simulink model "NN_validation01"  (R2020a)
settings: Solver=ode45  StartTime=0.0  StopTime=2000  RelTol=1e-3  EnableMultiTasking=on
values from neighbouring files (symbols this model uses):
  Ts = 0.2    [init_model.m]
libraries: neural x26

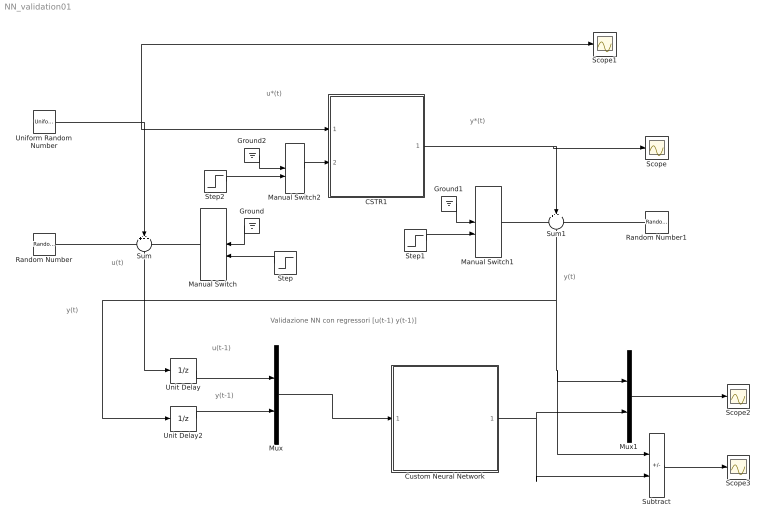
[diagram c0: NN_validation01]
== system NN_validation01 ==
  note: u(t)
  note: u*(t)
  note: y(t)
  note: y*(t)
  note: Validazione NN con regressori [u(t-1) y(t-1)]
  note: u(t-1)
  note: y(t)
  note: y(t-1)
  CSTR1 : Subsystem
  Custom Neural Network : Subsystem
      mask help: Custom Neural Network
  Ground : Ground
  Ground1 : Ground
  Ground2 : Ground
  Manual Switch : ManualSwitch
  Manual Switch1 : ManualSwitch
  Manual Switch2 : ManualSwitch
  Mux : Mux  Inputs=2
  Mux1 : Mux  Inputs=2
  Random Number : RandomNumber  Variance=0.0001  Seed=1  SampleTime=Ts
  Random Number1 : RandomNumber  Variance=0.0005  Seed=2  SampleTime=Ts
  Scope{,1..3} (4 alike) : Scope
  Step : Step  Time=1000  After=10  SampleTime=0
  Step1 : Step  Time=1000  After=10  SampleTime=0
  Step2 : Step  Time=1000  SampleTime=0
  Subtract : Sum  Inputs=+-
  Sum : Sum  Inputs=+++  SaturateOnIntegerOverflow=on
  Sum1 : Sum  Inputs=+++  SaturateOnIntegerOverflow=on
  Uniform Random Number : UniformRandomNumber  Minimum=0  Maximum=4  SampleTime=20
  Unit Delay : UnitDelay  SampleTime=Ts  HasFrameUpgradeWarning=on
  Unit Delay2 : UnitDelay  SampleTime=Ts  HasFrameUpgradeWarning=on
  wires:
  Uniform Random Number/1 -> CSTR1/1(w), Scope1/1, Sum/2
  Random Number/1 -> Sum/1
  Manual Switch/1 -> Sum/3
  Sum/1 -> Unit Delay/1
  Ground/1 -> Manual Switch/1
  Step/1 -> Manual Switch/2
  Ground1/1 -> Manual Switch1/1
  Step1/1 -> Manual Switch1/2
  CSTR1/1(Cb) -> Scope/1, Sum1/2
  Manual Switch1/1 -> Sum1/1
  Random Number1/1 -> Sum1/3
  Sum1/1 -> Subtract/1, Mux1/1, Unit Delay2/1
  Step2/1 -> Manual Switch2/2
  Manual Switch2/1 -> CSTR1/2(f)
  Ground2/1 -> Manual Switch2/1
  Unit Delay2/1 -> Mux/2
  Unit Delay/1 -> Mux/1
  Mux/1 -> Custom Neural Network/1(Input)
  Custom Neural Network/1(Output) -> Subtract/2, Mux1/2
  Mux1/1 -> Scope2/1
  Subtract/1 -> Scope3/1

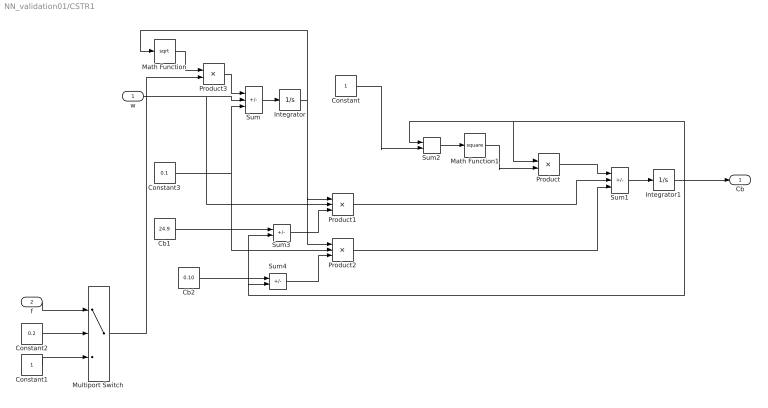
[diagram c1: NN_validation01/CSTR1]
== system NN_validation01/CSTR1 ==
  w : Inport
  f : Inport  Port=2
  Cb1 : Constant  Value=24.9
  Cb2 : Constant  Value=0.10
  Constant : Constant
  Constant1 : Constant
  Constant2 : Constant  Value=0.2
  Constant3 : Constant  Value=0.1
  Integrator : Integrator  InitialCondition=30  LimitOutput=on  LowerSaturationLimit=1
  Integrator1 : Integrator  InitialCondition=22
  Math Function : Math  Operator=sqrt
  Math Function1 : Math  Operator=square
  Multiport Switch : MultiPortSwitch  DataPortOrder=Zero-based contiguous  Inputs=2  zeroidx=on
  Product : Product  Inputs=*/  SaturateOnIntegerOverflow=on
  Product1 : Product  Inputs=/**  SaturateOnIntegerOverflow=on
  Product2 : Product  Inputs=/**  SaturateOnIntegerOverflow=on
  Product3 : Product
  Sum : Sum  Inputs=-++  SaturateOnIntegerOverflow=on
  Sum1 : Sum  Inputs=-++  SaturateOnIntegerOverflow=on
  Sum2 : Sum  SaturateOnIntegerOverflow=on
  Sum3 : Sum  Inputs=+-  SaturateOnIntegerOverflow=on
  Sum4 : Sum  Inputs=+-  SaturateOnIntegerOverflow=on
  Cb : Outport
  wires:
  Sum/1 -> Integrator/1
  Product3/1 -> Sum/1
  Math Function/1 -> Product3/1
  Integrator/1 -> Math Function/1, Product1/1, Product2/1
  Sum3/1 -> Product1/3
  Sum4/1 -> Product2/3
  Sum2/1 -> Math Function1/1
  Sum1/1 -> Integrator1/1
  Math Function1/1 -> Product/2
  Product/1 -> Sum1/1
  Product1/1 -> Sum1/2
  Product2/1 -> Sum1/3
  w/1 -> Sum/2, Product1/2
  Constant3/1 -> Product2/2, Sum/3
  Integrator1/1 -> Sum3/2, Sum4/2, Sum2/1, Product/1, Cb/1
  Constant1/1 -> Multiport Switch/3
  f/1 -> Multiport Switch/1
  Constant2/1 -> Multiport Switch/2
  Cb2/1 -> Sum4/1
  Cb1/1 -> Sum3/1
  Constant/1 -> Sum2/2
  Multiport Switch/1 -> Product3/2

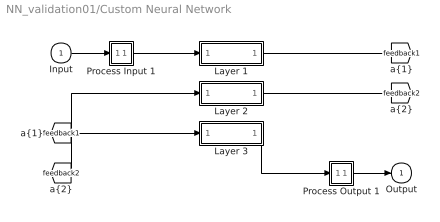
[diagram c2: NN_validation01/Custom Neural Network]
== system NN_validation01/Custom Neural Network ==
  Input : Inport  PortDimensions=2  SampleTime=0.2
  Layer 1 : Subsystem
  Layer 2 : Subsystem
  Layer 3 : Subsystem
  Process Input 1 : Subsystem
  Process Output 1 : Subsystem
  Output : Outport  InitialOutput=0
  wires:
  Input/1 -> Process Input 1/1(x)
  Process Output 1/1(y) -> Output/1
  Process Input 1/1(p) -> Layer 1/1("p{1}")
  Layer 1/1("a{1}") -> [feedback1]
  [feedback1] -> Layer 2/1("a{1} ")
  Layer 2/1("a{2}") -> [feedback2]
  [feedback2] -> Layer 3/1("a{2} ")
  Layer 3/1("a{3}") -> Process Output 1/1(a)

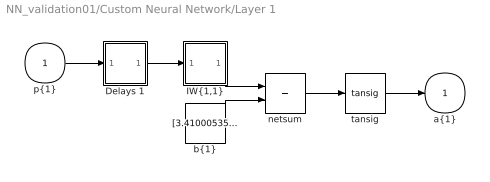
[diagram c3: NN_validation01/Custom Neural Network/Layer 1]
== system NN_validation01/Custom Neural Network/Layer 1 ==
  "p{1}" : Inport  PortDimensions=2  SampleTime=0.2
  Delays 1 : Subsystem
  "IW{1,1}" : Subsystem
  "b{1}" : Constant  Value=[3.410005357677003967609152823570184409618377685546875;3.968527131182099321193845753441564738750457763671875;-5.16528292497523811022119843983091413974761962890625;-2.98592875432198123775151543668471276760101318359375;-1.06890859356390865997354922001250088214874267578125;-2.854214797622984800540280048153363168239593505859375;-1.02557086847485212643960039713419973850250244140625]
  netsum : Sum  Inputs=2  InputSameDT=on  SaturateOnIntegerOverflow=on
  tansig : neural/Transfer Functions/tansig
  "a{1}" : Outport  InitialOutput=[0;0;0;0;0;0;0]
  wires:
  "p{1}"/1 -> Delays 1/1("p{1}")
  Delays 1/1("pd{1,1}") -> "IW{1,1}"/1("pd{1,1}")
  "IW{1,1}"/1("iz{1,1}") -> netsum/1
  "b{1}"/1 -> netsum/2
  netsum/1 -> tansig/1
  tansig/1 -> "a{1}"/1

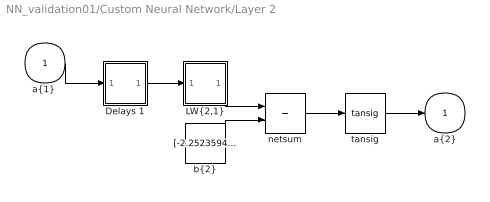
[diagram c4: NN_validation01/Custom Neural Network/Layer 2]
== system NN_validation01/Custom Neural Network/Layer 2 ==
  "a{1} " : Inport  PortDimensions=7  SampleTime=0.2
  Delays 1 : Subsystem
  "LW{2,1}" : Subsystem
  "b{2}" : Constant  Value=[-2.2523594995254239137238982948474586009979248046875;-0.50925995468204277027979287595371715724468231201171875;1.31533943350057658250307213165797293186187744140625;-1.8351214480429429709573696527513675391674041748046875;-1.7047429277987322659981828110176138579845428466796875;0.341559557754858300615552479939651675522327423095703125;-0.71047986742421820327564319086377508938312530517578125;-1.1423119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
  netsum : Sum  Inputs=2  InputSameDT=on  SaturateOnIntegerOverflow=on
  tansig : neural/Transfer Functions/tansig
  "a{2}" : Outport  InitialOutput=[0;0;0;0;0;0;0;0;0;0;0;0;0;0;0]
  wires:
  "a{1} "/1 -> Delays 1/1("p{2}")
  Delays 1/1("pd{2,1}") -> "LW{2,1}"/1("ad{2,1}")
  "LW{2,1}"/1("lz{2,1}") -> netsum/1
  "b{2}"/1 -> netsum/2
  netsum/1 -> tansig/1
  tansig/1 -> "a{2}"/1

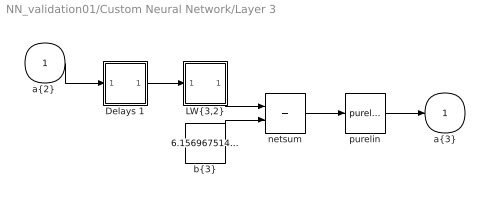
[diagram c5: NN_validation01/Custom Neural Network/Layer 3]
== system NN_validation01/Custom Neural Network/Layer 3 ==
  "a{2} " : Inport  PortDimensions=15  SampleTime=0.2
  Delays 1 : Subsystem
  "LW{3,2}" : Subsystem
  "b{3}" : Constant  Value=6.156967514716999545498765655793249607086181640625
  netsum : Sum  Inputs=2  InputSameDT=on  SaturateOnIntegerOverflow=on
  purelin : neural/Transfer Functions/purelin
  "a{3}" : Outport  InitialOutput=0
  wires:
  "a{2} "/1 -> Delays 1/1("p{3}")
  Delays 1/1("pd{3,2}") -> "LW{3,2}"/1("ad{3,2}")
  "LW{3,2}"/1("lz{3,2}") -> netsum/1
  "b{3}"/1 -> netsum/2
  netsum/1 -> purelin/1
  purelin/1 -> "a{3}"/1

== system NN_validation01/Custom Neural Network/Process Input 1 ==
  x : Inport  PortDimensions=2  SampleTime=0.2
  p : Outport  PortDimensions=2  SampleTime=0.2
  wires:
  x/1 -> p/1

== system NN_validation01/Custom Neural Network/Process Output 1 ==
  a : Inport  PortDimensions=1  SampleTime=0.2
  y : Outport  PortDimensions=1  SampleTime=0.2
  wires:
  a/1 -> y/1

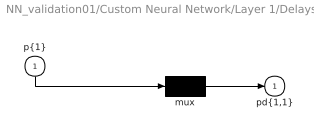
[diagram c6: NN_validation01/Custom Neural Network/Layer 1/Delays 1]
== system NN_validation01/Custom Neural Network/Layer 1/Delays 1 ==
  "p{1}" : Inport  PortDimensions=2  SampleTime=0.2
  mux : Mux  Inputs=1
  "pd{1,1}" : Outport
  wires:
  "p{1}"/1 -> mux/1
  mux/1 -> "pd{1,1}"/1

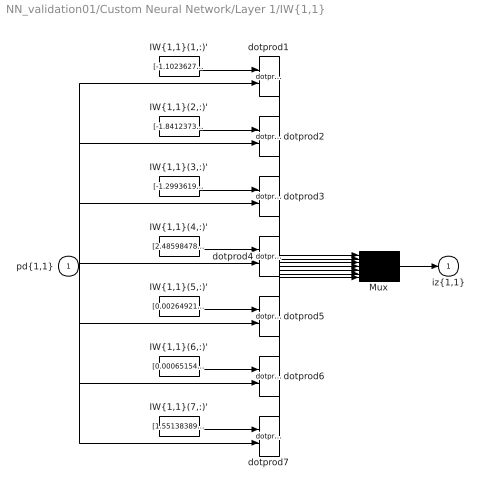
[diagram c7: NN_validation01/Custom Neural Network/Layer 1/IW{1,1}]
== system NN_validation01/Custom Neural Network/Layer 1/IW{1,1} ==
  "pd{1,1}" : Inport  PortDimensions=2  SampleTime=0.2
  "IW{1,1}(1,:)'" : Constant  Value=[-1.1023627620383342762266920544789172708988189697265625;0.73979188321445088494243691457086242735385894775390625]
  "IW{1,1}(2,:)'" : Constant  Value=[-1.8412373812163760344873253416153602302074432373046875;-0.80471225803352652850009008034248836338520050048828125]
  "IW{1,1}(3,:)'" : Constant  Value=[-1.299361926671609435146592659293673932552337646484375;-0.38777907964000235541135452876915223896503448486328125]
  "IW{1,1}(4,:)'" : Constant  Value=[2.485984782038082929744859939091838896274566650390625;-0.1401372905262729673392385620900313369929790496826171875]
  "IW{1,1}(5,:)'" : Constant  Value=[0.0026492101154049099535903177837781186099164187908172607421875;0.0895004498558449324008279290865175426006317138671875]
  "IW{1,1}(6,:)'" : Constant  Value=[0.000651547728287822126846950965273208566941320896148681640625;0.07858065504398224765392200197311467491090297698974609375]
  "IW{1,1}(7,:)'" : Constant  Value=[1.5513838905656138766886442681425251066684722900390625;-1.0120551416437333358544492512010037899017333984375]
  Mux : Mux  Inputs=7
  dotprod{1..7} (7 alike) : neural/Weight Functions/dotprod
  "iz{1,1}" : Outport
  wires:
  "IW{1,1}(1,:)'"/1 -> dotprod1/1
  "pd{1,1}"/1 -> dotprod1/2, dotprod2/2, dotprod3/2, dotprod4/2, dotprod5/2, dotprod6/2, dotprod7/2
  dotprod1/1 -> Mux/1
  "IW{1,1}(2,:)'"/1 -> dotprod2/1
  dotprod2/1 -> Mux/2
  "IW{1,1}(3,:)'"/1 -> dotprod3/1
  dotprod3/1 -> Mux/3
  "IW{1,1}(4,:)'"/1 -> dotprod4/1
  dotprod4/1 -> Mux/4
  "IW{1,1}(5,:)'"/1 -> dotprod5/1
  dotprod5/1 -> Mux/5
  "IW{1,1}(6,:)'"/1 -> dotprod6/1
  dotprod6/1 -> Mux/6
  "IW{1,1}(7,:)'"/1 -> dotprod7/1
  dotprod7/1 -> Mux/7
  Mux/1 -> "iz{1,1}"/1

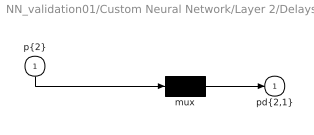
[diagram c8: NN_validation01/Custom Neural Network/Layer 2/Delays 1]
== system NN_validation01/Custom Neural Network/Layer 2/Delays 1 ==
  "p{2}" : Inport  PortDimensions=7  SampleTime=0.2
  mux : Mux  Inputs=1
  "pd{2,1}" : Outport
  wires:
  "p{2}"/1 -> mux/1
  mux/1 -> "pd{2,1}"/1

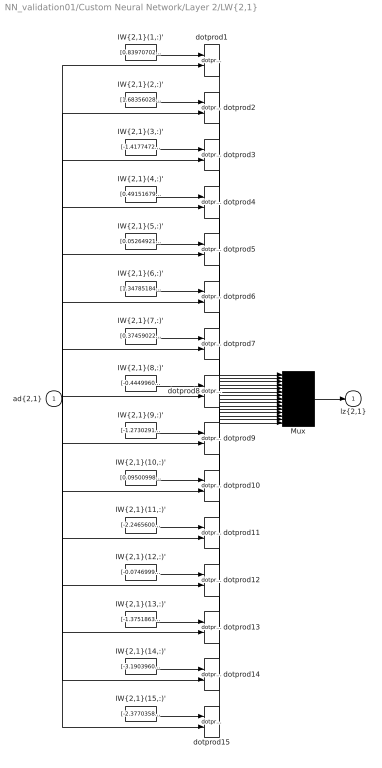
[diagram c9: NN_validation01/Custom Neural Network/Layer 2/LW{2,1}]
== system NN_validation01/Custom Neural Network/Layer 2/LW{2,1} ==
  "ad{2,1}" : Inport  PortDimensions=7  SampleTime=0.2
  "IW{2,1}(1,:)'" : Constant  Value=[0.839707029797628567990841474966146051883697509765625;-1.472141346293732500072337643359787762165069580078125;0.88689588741176639263841252613929100334644317626953125;0.3100104254000168868543596545350737869739532470703125;-2.348162079150298620078274325351230800151824951171875;3.312192265550647274352513704798184335231781005859375;3.0167591747950694980318075977265834808349609375]
  "IW{2,1}(10,:)'" : Constant  Value=[0.09500998862097996544573419441803707741200923919677734375;1.0922722336502646012235118178068660199642181396484375;0.33188497734036126463053051338647492229938507080078125;-0.0132476223515035351763202697839005850255489349365234375;-0.53564264209838763353133117561810649931430816650390625;2.71285895480330996321072234422899782657623291015625;-2.42010850150307543771077689598314464092254638671875]
  "IW{2,1}(11,:)'" : Constant  Value=[-2.2465600283505917644788496545515954494476318359375;0.307582595278991399734280776101513765752315521240234375;0.497451210795471332470896186350728385150432586669921875;1.0277839581201833052404026602744124829769134521484375;0.92315100856554155317468257635482586920261383056640625;-0.297887879916164888260965426525217480957508087158203125;0.1297665310981298281145512873990810476243495941162109375]
  "IW{2,1}(12,:)'" : Constant  Value=[-0.07469993825161669320777946268208324909210205078125;-0.1366089672588428893806877795213949866592884063720703125;-1.08813835281329485127344014472328126430511474609375;-2.687544894485628166336255162605084478855133056640625;-3.891996685481798667893826859653927385807037353515625;1.07362227069865667772319284267723560333251953125;-2.901033051576789478787077314336784183979034423828125]
  "IW{2,1}(13,:)'" : Constant  Value=[-1.37518635603682337631425980362109839916229248046875;0.0806749329025348849153687069701845757663249969482421875;-1.126932490567163380745796530391089618206024169921875;-0.368472092685779240017751590130501426756381988525390625;-1.7773338327356122956501849330379627645015716552734375;-0.2394194660186118872591265471783117391169071197509765625;1.271485640033413577754117795848287642002105712890625]
  "IW{2,1}(14,:)'" : Constant  Value=[-3.19039605253669211748501766123808920383453369140625;2.32007568201003078200983509304933249950408935546875;-1.2032141399369056244950115797109901905059814453125;1.072318296190253317234919450129382312297821044921875;-0.282781820437841779902754524300689809024333953857421875;-3.153015872697419563763787664356641471385955810546875;0.7367047677992195620078064166591502726078033447265625]
  "IW{2,1}(15,:)'" : Constant  Value=[-2.37703589289161687503337816451676189899444580078125;-0.252866282843091483290010046403040178120136260986328125;-0.54884116877321786898136224408517591655254364013671875;-0.37299496370290385893753182244836352765560150146484375;-0.37781382582181788354347418135148473083972930908203125;1.049624366726357838075500694685615599155426025390625;2.22865752576128794970600210945121943950653076171875]
  "IW{2,1}(2,:)'" : Constant  Value=[1.6835602843496244584997612037113867700099945068359375;1.37767858546537436126300235628150403499603271484375;-1.25578785825161265421456846524961292743682861328125;0.0025934453807945380410249214264695183373987674713134765625;-3.774935288732403027012196616851724684238433837890625;-1.6230533969681264494511196971870958805084228515625;-0.09129736775341044940912382799069746397435665130615234375]
  "IW{2,1}(3,:)'" : Constant  Value=[-1.4177472765446783586895662665483541786670684814453125;3.87102870440241719762752836686559021472930908203125;0.434976128739432255088104284368455410003662109375;1.996505223764537984010303262039087712764739990234375;1.9365670899909284141671150791808031499385833740234375;-4.8345064843095588713595134322531521320343017578125;-2.88421897567884055746390004060231149196624755859375]
  "IW{2,1}(4,:)'" : Constant  Value=[0.491516795819420482249739734470495022833347320556640625;-0.97015295368330989322913637806777842342853546142578125;-1.6461577736956989337357981639797799289226531982421875;-0.02368795477953096473289207324341987259685993194580078125;1.3496939712894924223718362554791383445262908935546875;0.749904211023995959095600483124144375324249267578125;-1.13394981045262621677238712436519563198089599609375]
  "IW{2,1}(5,:)'" : Constant  Value=[0.0526492105191031789512834393462981097400188446044921875;-0.70801550160030546354761327165761031210422515869140625;-3.9506603848980024196180238504894077777862548828125;-2.473846049632155708053460330120287835597991943359375;0.1192687936217095845403690645980532281100749969482421875;-1.729683349811485637559371753013692796230316162109375;-1.1762801585132347526041485252790153026580810546875]
  "IW{2,1}(6,:)'" : Constant  Value=[1.3478518425068901631647122485446743667125701904296875;-2.39781466117784614056063219322822988033294677734375;0.05306427218267552314845403316212468780577182769775390625;0.18935753028191271152280705791781656444072723388671875;2.469774191732282186961811021319590508937835693359375;-0.8294247869117958860130102038965560495853424072265625;-0.468548041328876341271580940883723087608814239501953125]
  "IW{2,1}(7,:)'" : Constant  Value=[0.374590228792672730318003004867932759225368499755859375;0.7179497175763887018007380902417935431003570556640625;-0.331804513263293798797093359098653309047222137451171875;-0.000682635994757380647202094081649192958138883113861083984375;-1.0744419663733688619089434723719023168087005615234375;-3.530508381544886997716048426809720695018768310546875;0.8497530070893082321248357402510009706020355224609375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
  "IW{2,1}(8,:)'" : Constant  Value=[-0.444996005783854453596859457320533692836761474609375;-4.74590578428593179438621518784202635288238525390625;-1.2469535545989052227611182388500310480594635009765625;-2.03426991407743340545266619301401078701019287109375;-2.646009358020870561034598722471855580806732177734375;5.1060911129817352360760196461342275142669677734375;2.1435860869179492738112458027899265289306640625]
  "IW{2,1}(9,:)'" : Constant  Value=[-1.2730291895642409372157999314367771148681640625;1.0490289390464810903580428202985785901546478271484375;-0.83363923174218668155077693882049061357975006103515625;1.1237536104988470331278449521050788462162017822265625;-0.60602322014761356161471894665737636387348175048828125;-0.61712778802297874047866343971691094338893890380859375;0.74847970692010978854824543304857797920703887939453125]
  Mux : Mux  Inputs=15
  dotprod{1..15} (15 alike) : neural/Weight Functions/dotprod
  "lz{2,1}" : Outport
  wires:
  "IW{2,1}(1,:)'"/1 -> dotprod1/1
  "ad{2,1}"/1 -> dotprod1/2, dotprod2/2, dotprod3/2, dotprod4/2, dotprod5/2, dotprod6/2, dotprod7/2, dotprod8/2, dotprod9/2, dotprod10/2, dotprod11/2, dotprod12/2, dotprod13/2, dotprod14/2, dotprod15/2
  dotprod1/1 -> Mux/1
  "IW{2,1}(2,:)'"/1 -> dotprod2/1
  dotprod2/1 -> Mux/2
  "IW{2,1}(3,:)'"/1 -> dotprod3/1
  dotprod3/1 -> Mux/3
  "IW{2,1}(4,:)'"/1 -> dotprod4/1
  dotprod4/1 -> Mux/4
  "IW{2,1}(5,:)'"/1 -> dotprod5/1
  dotprod5/1 -> Mux/5
  "IW{2,1}(6,:)'"/1 -> dotprod6/1
  dotprod6/1 -> Mux/6
  "IW{2,1}(7,:)'"/1 -> dotprod7/1
  dotprod7/1 -> Mux/7
  "IW{2,1}(8,:)'"/1 -> dotprod8/1
  dotprod8/1 -> Mux/8
  "IW{2,1}(9,:)'"/1 -> dotprod9/1
  dotprod9/1 -> Mux/9
  "IW{2,1}(10,:)'"/1 -> dotprod10/1
  dotprod10/1 -> Mux/10
  "IW{2,1}(11,:)'"/1 -> dotprod11/1
  dotprod11/1 -> Mux/11
  "IW{2,1}(12,:)'"/1 -> dotprod12/1
  dotprod12/1 -> Mux/12
  "IW{2,1}(13,:)'"/1 -> dotprod13/1
  dotprod13/1 -> Mux/13
  "IW{2,1}(14,:)'"/1 -> dotprod14/1
  dotprod14/1 -> Mux/14
  "IW{2,1}(15,:)'"/1 -> dotprod15/1
  dotprod15/1 -> Mux/15
  Mux/1 -> "lz{2,1}"/1

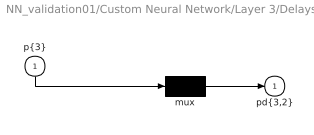
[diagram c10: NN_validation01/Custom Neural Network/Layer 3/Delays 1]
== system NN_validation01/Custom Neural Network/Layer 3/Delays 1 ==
  "p{3}" : Inport  PortDimensions=15  SampleTime=0.2
  mux : Mux  Inputs=1
  "pd{3,2}" : Outport
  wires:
  "p{3}"/1 -> mux/1
  mux/1 -> "pd{3,2}"/1

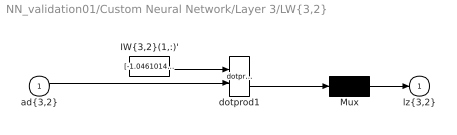
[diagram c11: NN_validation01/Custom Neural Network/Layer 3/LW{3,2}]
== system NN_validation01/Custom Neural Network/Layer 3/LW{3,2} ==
  "ad{3,2}" : Inport  PortDimensions=15  SampleTime=0.2
  "IW{3,2}(1,:)'" : Constant  Value=[-1.046101461144682165382846505963243544101715087890625;-2.769137531128453844075920642353594303131103515625;2.668199693128057159441368639818392693996429443359375;-0.77282167375571508838305589961237274110317230224609375;-2.19217601037632281446576598682440817356109619140625;0.287365691903721576228036838074331171810626983642578125;-3.669643383232441546937252496718429028987884521484375;2.5933077992477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
  Mux : Mux  Inputs=1
  dotprod1 : neural/Weight Functions/dotprod
  "lz{3,2}" : Outport
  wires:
  "IW{3,2}(1,:)'"/1 -> dotprod1/1
  "ad{3,2}"/1 -> dotprod1/2
  dotprod1/1 -> Mux/1
  Mux/1 -> "lz{3,2}"/1
